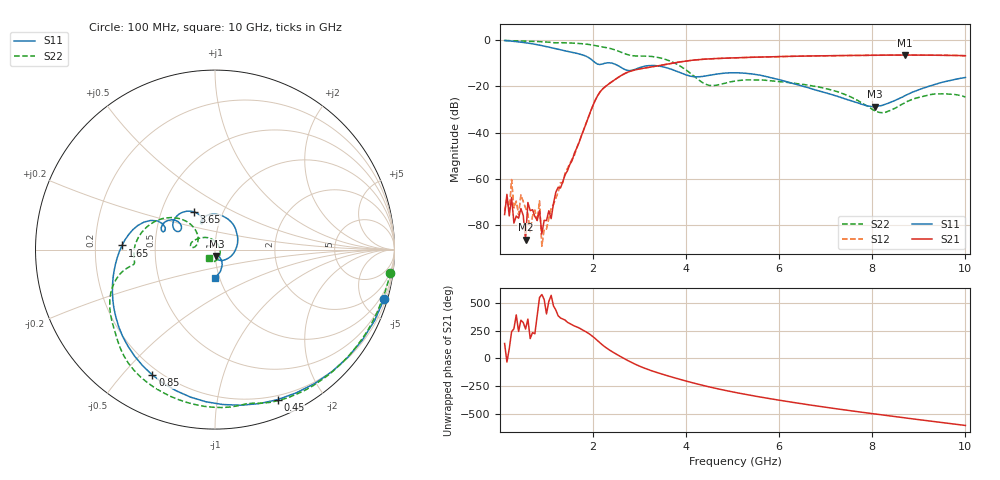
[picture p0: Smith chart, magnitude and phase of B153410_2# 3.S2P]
!  2-Port S-parameters saved by WinCal
! VAR MeasName=S-Parameters (CALIBRATED_DATA) read from VNA (N5245A)
! VAR MeasDate=2016-12-23 9:59:30
! VAR NAME=B153410_2# 3
! VAR FILENAME=B153410_2# 3.S2P
! VAR DATE=2016-12-23 9:59:30
! VAR PHYS_PORTS=1,2
# Hz S DB R 50
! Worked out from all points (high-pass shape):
!   199 points, 100 MHz to 10 GHz, reference 50 ohm
!   highest |S21| = -6.42 dB at 8.7 GHz (marker M1); lowest = -86.2 dB at 550 MHz (marker M2)
!   |S21| within 3 dB of the highest: 3.863 GHz to end of sweep
!   lowest |S11| = -28.8 dB at 8.05 GHz (marker M3), VSWR 1.08, Z = 50.7 - j3.61 ohm
!   |S11| at or under -10 dB: 2.069 GHz to 2.252 GHz (183 MHz wide, 8.47 % of centre); 2.416 GHz to end of sweep
!   |S22| runs from -31.4 to -0.1 dB; largest |S21 - S12| = 0.0027
!   S11 on the Smith chart (normalised r, x): 100 MHz: 0.46, -7.00; 450 MHz: 0.16, -1.49; 850 MHz: 0.17, -0.61; 1.65 GHz: 0.32, +0.02; 3.65 GHz: 0.73, +0.33; 10 GHz: 0.95, -0.30
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1e8  -0.16 -16.2  -75.39 133.4  -74.04 -136.2  -0.13 -7.5
1.5e8  -0.24 -24.0  -66.65 -34.1  -68.25 52.8  -0.17 -10.9
2e8  -0.32 -31.5  -75.98 86.3  -73.75 99.4  -0.21 -14.2
2.5e8  -0.42 -39.0  -67.96 -119.8  -60.26 -96.7  -0.25 -17.6
3e8  -0.52 -46.3  -79.08 -93.5  -72.54 -7.3  -0.28 -21.0
4.5e8  -0.86 -67.3  -72.81 -16.5  -66.84 40.0  -0.36 -30.9
5.5e8  -1.12 -80.7  -86.21 -95.9  -72.51 114.6  -0.42 -37.5
6e8  -1.27 -87.1  -70.19 -5.8  -74.99 142.5  -0.45 -40.8
8e8  -1.95 -111.0  -77.87 22.3  -78.00 -111.0  -0.59 -53.9
8.5e8  -2.15 -116.6  -73.63 -172.0  -69.46 81.5  -0.63 -57.2
1e9  -2.80 -131.9  -77.96 40.4  -81.63 -66.7  -0.79 -67.1
1.65e9  -5.70 177.5  -46.62 -76.8  -46.65 -80.3  -1.37 -106.9
1.75e9  -6.23 170.1  -41.30 -97.6  -41.29 -98.3  -1.52 -113.5
2.25e9  -10.01 160.5  -20.30 104.6  -20.26 104.9  -3.11 -145.2
3.4e9  -11.13 132.3  -11.09 -132.1  -11.07 -132.2  -7.49 167.7
3.65e9  -12.36 119.1  -10.16 -164.0  -10.16 -164.2  -8.98 152.3
5.05e9  -14.09 93.0  -7.63 52.2  -7.65 52.2  -17.66 174.2
6.7e9  -21.03 -32.5  -6.81 -63.8  -6.82 -63.7  -19.71 140.9
8.05e9  -28.76 -77.4  -6.49 -142.3  -6.49 -142.3  -30.52 50.0
8.35e9  -27.23 -62.4  -6.47 -158.8  -6.45 -158.7  -30.62 -10.3
8.7e9  -24.02 -58.4  -6.42 -177.9  -6.43 -177.8  -27.09 -56.3
1e10  -16.10 -90.6  -6.73 113.8  -6.71 114.0  -24.61 -127.7
